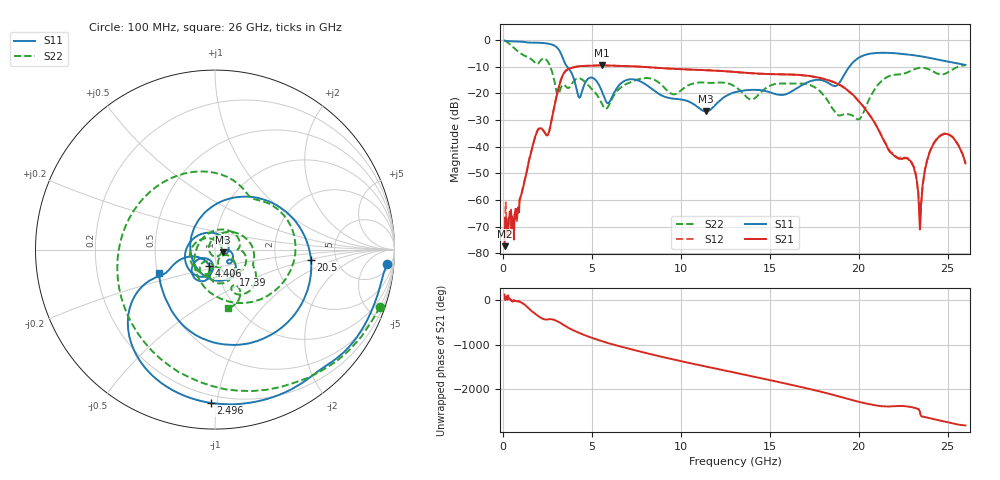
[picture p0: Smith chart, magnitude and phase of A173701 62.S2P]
!  2-Port S-parameters saved by WinCal
! VAR MeasName=S-Parameters (CALIBRATED_DATA) read from VNA (N5245A)
! VAR MeasDate=2017-6-7 10:32:33
! VAR NAME=A173701 62
! VAR FILENAME=A173701 62.S2P
! VAR DATE=2017-6-7 10:32:33
! VAR PHYS_PORTS=1,2
# Hz S DB R 50
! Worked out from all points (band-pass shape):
!   801 points, 100 MHz to 26 GHz, reference 50 ohm
!   highest |S21| = -9.55 dB at 5.571 GHz (marker M1); lowest = -77.3 dB at 100 MHz (marker M2)
!   |S21| within 3 dB of the highest: 3.427 GHz to 14.12 GHz (10.69 GHz wide, 122 % of centre); 14.12028 GHz to 14.15867 GHz (38.39 MHz wide, 0.272 % of centre)
!   lowest |S11| = -26.8 dB at 11.4 GHz (marker M3), VSWR 1.10, Z = 54.5 - j1.62 ohm
!   |S11| at or under -10 dB: 3.61 GHz to 19.49 GHz (15.88 GHz wide, 137 % of centre)
!   |S22| runs from -29.8 to -0.2 dB; largest |S21 - S12| = 0.004
!   S11 on the Smith chart (normalised r, x): 100 MHz: 9, -20; 2.496 GHz: 0.15, -0.96; 4.406 GHz: 0.92, -0.17; 17.39 GHz: 1.18, -0.34; 20.5 GHz: 3.23, -0.52; 26 GHz: 0.51, -0.15
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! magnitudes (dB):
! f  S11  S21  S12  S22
! 100 MHz  -0.3  -77.3  -72.7  -0.2
! 747.5 MHz  -0.6  -63.4  -64.7  -3.8
! 1.913 GHz  -1.1  -34.5  -34.5  -9.1
! 2.496 GHz  -1.4  -35.8  -35.7  -7.9
! 3.079 GHz  -3.1  -19.5  -19.5  -20.6
! 3.402 GHz  -7.4  -12.8  -12.8  -16.8
! 4.406 GHz  -20.3  -9.8  -9.8  -14.7
! 4.438 GHz  -19.6  -9.8  -9.8  -14.8
! 4.956 GHz  -14.1  -9.7  -9.7  -18.1
! 5.571 GHz  -19.3  -9.5  -9.6  -24.0
! 8.744 GHz  -20.1  -10.5  -10.5  -15.9
! 11.4 GHz  -26.8  -11.4  -11.4  -16.0
! 13.05 GHz  -19.6  -12.0  -12.0  -17.5
! 17.39 GHz  -15.3  -13.8  -13.7  -17.3
! 18.88 GHz  -16.4  -16.7  -16.7  -28.3
! 20.5 GHz  -5.4  -27.1  -27.1  -23.6
! 21.69 GHz  -4.9  -41.4  -41.1  -13.6
! 22.99 GHz  -5.7  -46.3  -45.9  -11.4
! 23.44 GHz  -6.1  -71.1  -68.9  -10.5
! 23.9 GHz  -6.6  -44.1  -44.0  -10.9
! 24.51 GHz  -7.5  -36.3  -36.3  -12.9
! 26 GHz  -9.4  -46.3  -46.1  -9.5
